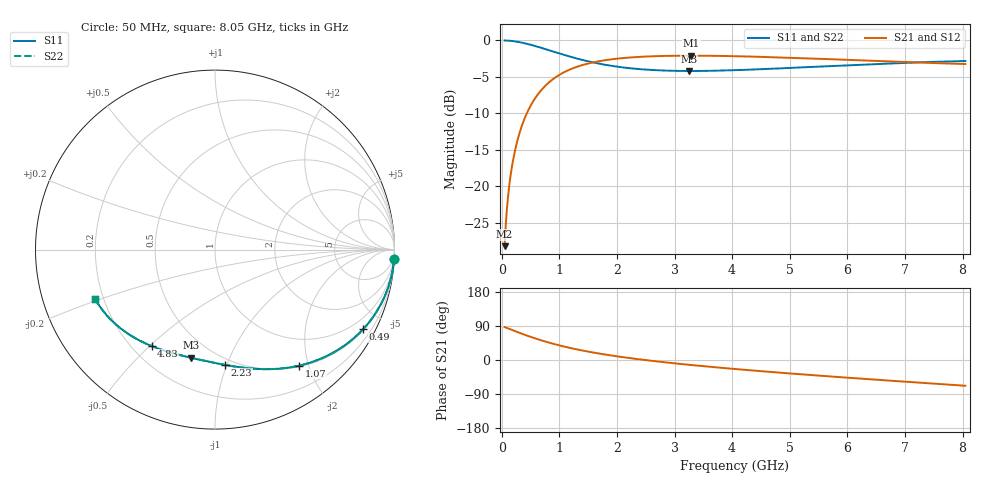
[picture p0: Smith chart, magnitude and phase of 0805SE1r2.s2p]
! AVX Thin Film Operation		Date: August 2001
! Description: Accu-P® Series, Thin Film, SMD, RF Capacitor
! Part Number: 08051J1R2ABT
! 50 MHz  -  8.05 GHz
! Serial Measurements
# mhz S db R 50
!	S11		S21		S12		S22
!	dB	Phase	dB	Phase	dB	Phase	dB	Phase
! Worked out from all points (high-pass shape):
!   401 points, 50 MHz to 8.05 GHz, reference 50 ohm
!   highest |S21| = -2.09 dB at 3.29 GHz (marker M1); lowest = -28.2 dB at 50 MHz (marker M2)
!   |S21| within 3 dB of the highest: 928.4 MHz to end of sweep
!   lowest |S11| = -4.2 dB at 3.25 GHz (marker M3), VSWR 4.23, Z = 18.8 - j36.5 ohm
!   |S11| at or under -10 dB: nowhere
!   |S22| runs from -4.2 to 0.0 dB; largest |S21 - S12| = 0
!   S11 on the Smith chart (normalised r, x): 50 MHz: 1, -38; 490 MHz: 0.54, -3.89; 1.07 GHz: 0.52, -1.85; 2.23 GHz: 0.45, -0.98; 4.83 GHz: 0.28, -0.51; 8.05 GHz: 0.17, -0.19
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50  -0.01 -3.0  -28.19 87.0  -28.19 87.0  -0.01 -3.0
70  -0.01 -4.2  -25.27 85.8  -25.27 85.8  -0.01 -4.2
130  -0.04 -7.9  -19.94 82.1  -19.94 82.1  -0.04 -7.9
170  -0.07 -10.3  -17.65 79.7  -17.65 79.7  -0.07 -10.3
210  -0.11 -12.6  -15.86 77.4  -15.86 77.4  -0.11 -12.6
270  -0.19 -16.1  -13.78 73.9  -13.78 73.9  -0.19 -16.1
330  -0.27 -19.6  -12.15 70.4  -12.15 70.4  -0.27 -19.6
490  -0.57 -28.3  -9.12 61.7  -9.12 61.7  -0.57 -28.3
610  -0.83 -34.4  -7.58 55.6  -7.58 55.6  -0.83 -34.4
750  -1.17 -41.0  -6.27 48.9  -6.27 48.9  -1.17 -41.0
1070  -1.95 -54.1  -4.41 35.9  -4.41 35.9  -1.95 -54.1
1390  -2.65 -64.7  -3.40 25.3  -3.40 25.3  -2.65 -64.7
1790  -3.33 -75.4  -2.72 14.5  -2.72 14.5  -3.33 -75.4
2230  -3.81 -85.1  -2.34 4.9  -2.34 4.9  -3.81 -85.1
2730  -4.10 -94.3  -2.15 -4.3  -2.15 -4.3  -4.10 -94.3
3250  -4.19 -102.6  -2.09 -12.6  -2.09 -12.6  -4.19 -102.6
3290  -4.19 -103.2  -2.09 -13.2  -2.09 -13.2  -4.19 -103.2
4050  -4.08 -113.7  -2.16 -23.8  -2.16 -23.8  -4.08 -113.7
4830  -3.83 -123.4  -2.33 -33.4  -2.33 -33.4  -3.83 -123.4
5390  -3.63 -129.8  -2.48 -39.9  -2.48 -39.9  -3.63 -129.8
6730  -3.16 -144.3  -2.89 -54.4  -2.89 -54.4  -3.16 -144.3
8050  -2.82 -157.8  -3.24 -68.0  -3.24 -68.0  -2.82 -157.8
